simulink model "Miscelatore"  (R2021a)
settings: Solver=VariableStepAuto  StartTime=0.0  StopTime=10000  MaxStep=1  RelTol=1e-3
undefined symbols (not defined in the file or in its folder): A, cv, cvm, h, Mm, P, rho, Rma, T0, T1star, T2star, Tamb, Tm0, w1star, w2star, wstar, z0

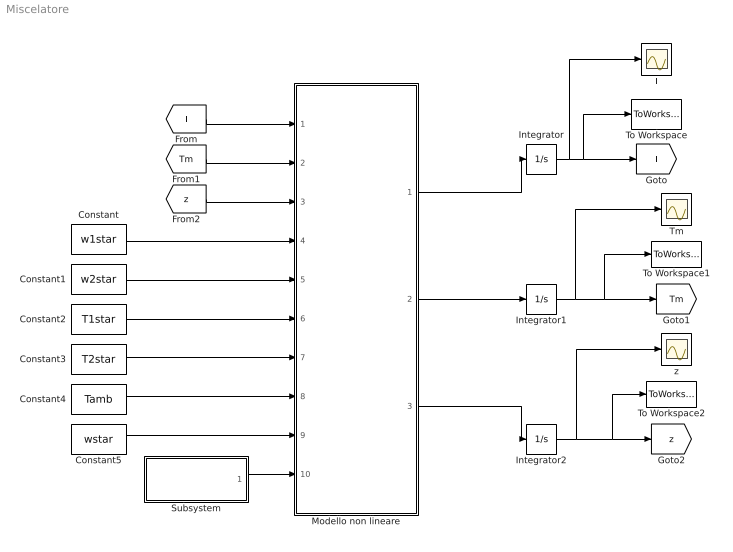
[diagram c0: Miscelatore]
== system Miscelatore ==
  Constant : Constant  Value=w1star
  Constant1 : Constant  Value=w2star
  Constant2 : Constant  Value=T1star
  Constant3 : Constant  Value=T2star
  Constant4 : Constant  Value=Tamb
  Constant5 : Constant  Value=wstar
  Integrator : Integrator  InitialCondition=T0
  Integrator1 : Integrator  InitialCondition=Tm0
  Integrator2 : Integrator  InitialCondition=z0
  Modello non lineare : MATLAB Function  TreatAsAtomicUnit=on
  Subsystem : Subsystem
  T : Scope
  Tm : Scope
  To Workspace : ToWorkspace  VariableName=T  SaveFormat=Timeseries  SampleTime=-1
  To Workspace1 : ToWorkspace  VariableName=Tm  SaveFormat=Timeseries  SampleTime=-1
  To Workspace2 : ToWorkspace  VariableName=z  SaveFormat=Timeseries  SampleTime=-1
  z : Scope
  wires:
  Modello non lineare/1(Tdot) -> Integrator/1
  Modello non lineare/2(Tmdot) -> Integrator1/1
  Modello non lineare/3(zdot) -> Integrator2/1
  Integrator/1 -> T/1, To Workspace/1, [T]
  Integrator1/1 -> Tm/1, To Workspace1/1, [Tm]
  Integrator2/1 -> z/1, To Workspace2/1, [z]
  [T] -> Modello non lineare/1(T)
  [Tm] -> Modello non lineare/2(Tm)
  [z] -> Modello non lineare/3(z)
  Subsystem/1(par) -> Modello non lineare/10(par)
  Constant/1 -> Modello non lineare/4(w1)
  Constant1/1 -> Modello non lineare/5(w2)
  Constant2/1 -> Modello non lineare/6(T1)
  Constant3/1 -> Modello non lineare/7(T2)
  Constant4/1 -> Modello non lineare/8(Tamb)
  Constant5/1 -> Modello non lineare/9(w)

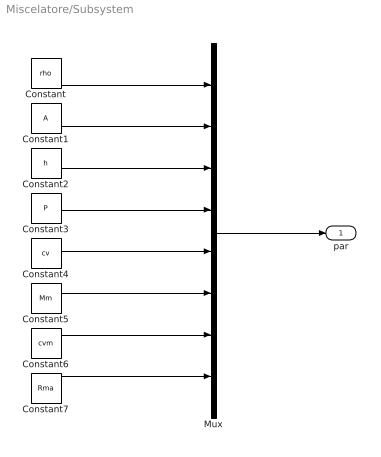
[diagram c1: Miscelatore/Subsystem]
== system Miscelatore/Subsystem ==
  Constant : Constant  Value=rho
  Constant1 : Constant  Value=A
  Constant2 : Constant  Value=h
  Constant3 : Constant  Value=P
  Constant4 : Constant  Value=cv
  Constant5 : Constant  Value=Mm
  Constant6 : Constant  Value=cvm
  Constant7 : Constant  Value=Rma
  Mux : Mux  Inputs=8
  par : Outport
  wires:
  Constant/1 -> Mux/1
  Constant1/1 -> Mux/2
  Constant2/1 -> Mux/3
  Constant3/1 -> Mux/4
  Constant4/1 -> Mux/5
  Constant5/1 -> Mux/6
  Constant6/1 -> Mux/7
  Constant7/1 -> Mux/8
  Mux/1 -> par/1

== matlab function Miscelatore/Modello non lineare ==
function [Tdot,Tmdot,zdot] = Miscelatore(T,Tm,z,w1,w2,T1,T2,Tamb,w,par)

rho=par(1);
A=par(2);
h=par(3);
P=par(4);
cv=par(5);
Mm=par(6);
cvm=par(7);
Rma=par(8);


Tdot=-((w1+w2)/(rho*A*z)+h*P/(rho*cv*A))*T+h*P/(rho*cv*A)*Tm+w1*T1/(rho*A*z)+w2*T2/(rho*A*z);

Tmdot=-(h*P*z/(Mm*cvm)+1/(Mm*cvm*Rma))*Tm+h*P*z/(Mm*cvm)*T+Tamb/(Mm*cvm*Rma);

zdot=(w1+w2-w)/(rho*A);
